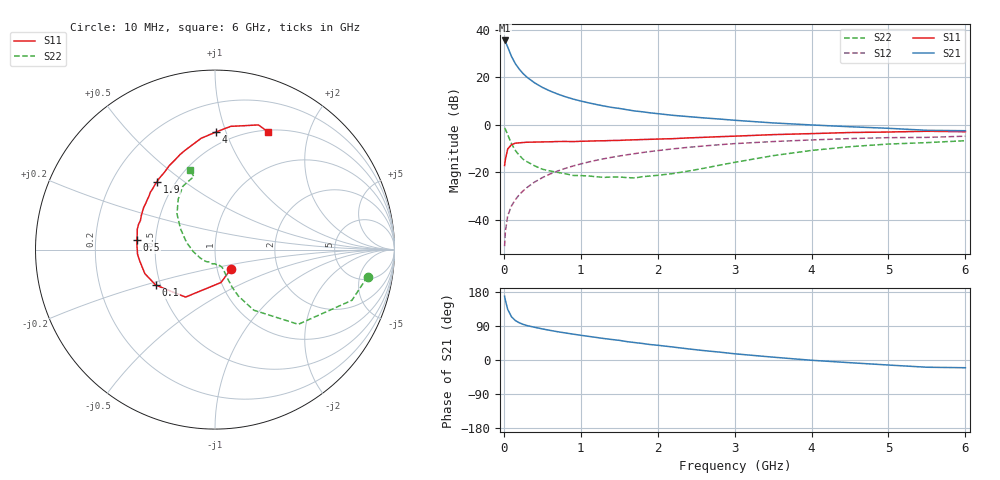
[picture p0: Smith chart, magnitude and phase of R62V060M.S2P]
! SIEMENS Small Signal Semiconductors
! BFR193
! Si NPN RF Bipolar Junction Transistor in SOT23
! VCE = 2 V  IC = 60 mA
! Common Emitter S-Parameters:  May  1996
# GHz  S  MA  R  50
!  f  S11  S21  S12  S22
! GHz  MAG  ANG  MAG  ANG  MAG  ANG  MAG  ANG
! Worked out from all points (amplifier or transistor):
!   36 points, 10 MHz to 6 GHz, reference 50 ohm
!   highest |S21| = 35.6 dB at 10 MHz (marker M1)
!   |S21| within 3 dB of that: start of sweep to 52.93 MHz
!   unconditionally stable (mu >= 1): 274.5 MHz to 2.091 GHz
!   at 250 MHz: K = 0.99, MSG = 24.7 dB, |S12| = -27.8 dB
!   at 1.4 GHz: K = 1.03, MAG = 9.5 dB, |S12| = -13.6 dB
!   at 6 GHz: K = 0.97, MSG = 1.1 dB, |S12| = -4.7 dB
!   S11 on the Smith chart (normalised r, x): 10 MHz: 1.16, -0.26; 100 MHz: 0.47, -0.22; 500 MHz: 0.39, +0.05; 1.9 GHz: 0.40, +0.40; 4 GHz: 0.40, +0.93; 6 GHz: 0.52, +1.41
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0.01  0.1401 -50.8  60.06 168.3  0.0028 81.0  0.8634 -10.0
0.02  0.1864 -79.7  56.96 157.4  0.0057 80.7  0.8137 -20.3
0.05  0.3113 -121.8  43.68 133.6  0.0122 70.6  0.6234 -41.9
0.1  0.3849 -149.1  27.58 114.0  0.0198 70.9  0.4006 -57.4
0.15  0.4132 -161.1  19.46 104.0  0.0267 71.3  0.2891 -63.3
0.2  0.4194 -168.4  14.98 98.3  0.0339 73.3  0.2298 -65.5
0.25  0.426 -172.5  12.07 94.1  0.0408 74.4  0.1896 -66.2
0.3  0.4324 -176.8  10.14 90.9  0.048 75.2  0.1685 -66.5
0.4  0.435 177.3  7.694 86.3  0.0628 75.2  0.1375 -67.0
0.5  0.4392 173.1  6.179 82.1  0.0775 75.1  0.117 -66.9
0.6  0.4412 169.2  5.186 78.2  0.0924 73.9  0.1073 -68.3
0.7  0.4475 165.4  4.469 74.6  0.1071 73.0  0.1002 -70.0
0.8  0.4486 161.7  3.921 71.4  0.1218 71.6  0.0938 -73.6
1.1  0.4564 152.3  2.922 62.4  0.1655 67.5  0.0843 -83.4
1.4  0.4699 142.9  2.342 54.2  0.2079 63.0  0.0802 -97.0
1.9  0.4976 130.5  1.798 40.8  0.2751 55.2  0.084 -130.7
2.2  0.5139 123.5  1.592 34.2  0.3135 50.3  0.0946 -150.4
3.5  0.6249 97.1  1.102 7.5  0.4467 29.0  0.2254 148.7
4  0.6564 89.3  0.999 -0.7  0.4832 21.8  0.2904 136.8
4.5  0.6923 82.7  0.916 -7.1  0.5156 14.7  0.3483 126.0
5.5  0.7357 70.8  0.77 -19.1  0.5464 1.0  0.4242 106.1
6  0.7193 65.8  0.755 -20.4  0.5795 -3.0  0.4653 107.6
